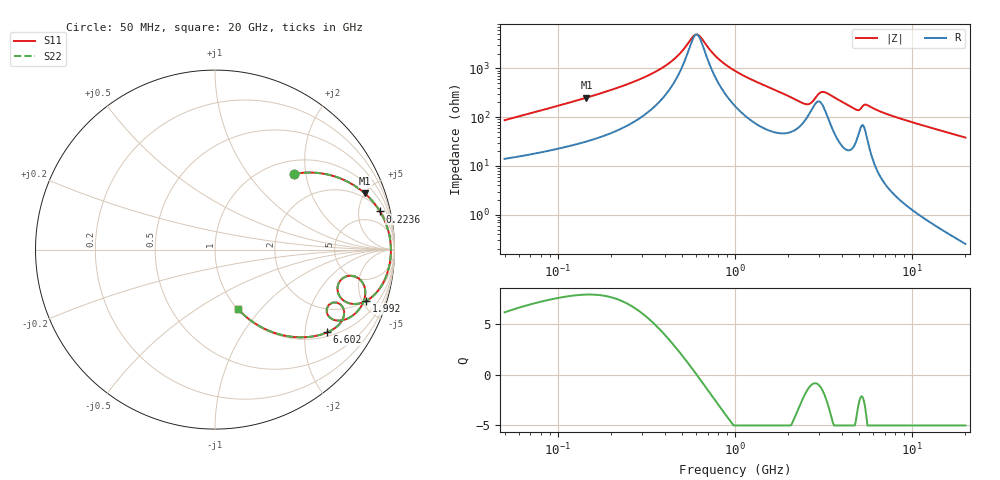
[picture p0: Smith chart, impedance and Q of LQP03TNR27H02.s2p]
!Murata Part Number: LQP03TNR27H02
!These Parameters are Measured in Series Mode Connection
!  o--[Z]--o
!Port1  Port2
!  o-------o
!Freq. Start=50[MHz] Stop=20[GHz], 401[Steps]
# Hz S RI R 50
!Freq.(Hz) S11(Real) S11(Imag) S21(Real) S21(Imag) S12(Real) S12(Imag) S22(Real) S22(Imag)
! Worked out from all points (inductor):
!   401 points, 50 MHz to 20 GHz, reference 50 ohm
!   read as one part in series: L = 268 nH near 51.52 MHz
!   highest Q = 7.85 at 144.8 MHz (marker M1), where L = 273 nH
!   self-resonance near 606.3 MHz
!   S11 on the Smith chart (normalised r, x): 50 MHz: 1.28, +1.71; 223.6 MHz: 2.13, +8.23; 1.992 GHz: 1.95, -5.37; 6.602 GHz: 1.12, -2.61; 20 GHz: 1.01, -0.76
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5e7  0.4391 0.4211  0.5609 -0.4211  0.5609 -0.4211  0.4391 0.4211
1.364002e8  0.8178 0.3274  0.1822 -0.3274  0.1822 -0.3274  0.8178 0.3274
1.448224e8  0.8337 0.3141  0.1663 -0.3141  0.1663 -0.3141  0.8337 0.3141
2.236068e8  0.9193 0.2124  0.0807 -0.2124  0.0807 -0.2124  0.9193 0.2124
3.721004e8  0.9672 0.0989  0.0328 -0.0989  0.0328 -0.0989  0.9672 0.0989
4.589149e8  0.9758 0.0558  0.0242 -0.0558  0.0242 -0.0558  0.9758 0.0558
6.100003e8  0.9802 -0.00121  0.0198 0.00121  0.0198 0.00121  0.9802 -0.00121
7.987718e8  0.9769 -0.0561  0.0231 0.0561  0.0231 0.0561  0.9769 -0.0561
1e9  0.9676 -0.1049  0.0324 0.1049  0.0324 0.1049  0.9676 -0.1049
1.99176e9  0.8429 -0.2858  0.1571 0.2858  0.1571 0.2858  0.8429 -0.2858
2.419936e9  0.7176 -0.2846  0.2824 0.2846  0.2824 0.2846  0.7176 -0.2846
2.728004e9  0.6972 -0.1736  0.3028 0.1736  0.3028 0.1736  0.6972 -0.1736
3.121702e9  0.8199 -0.1806  0.1801 0.1806  0.1801 0.1806  0.8199 -0.1806
3.680849e9  0.8206 -0.3052  0.1794 0.3052  0.1794 0.3052  0.8206 -0.3052
4.539627e9  0.6996 -0.3952  0.3004 0.3952  0.3004 0.3952  0.6996 -0.3952
4.966507e9  0.6226 -0.3493  0.3774 0.3493  0.3774 0.3493  0.6226 -0.3493
5.273168e9  0.6793 -0.295  0.3207 0.295  0.3207 0.295  0.6793 -0.295
5.683258e9  0.7154 -0.3782  0.2846 0.3782  0.2846 0.3782  0.7154 -0.3782
6.601595e9  0.6255 -0.4611  0.3745 0.4611  0.3745 0.4611  0.6255 -0.4611
7.442007e9  0.5512 -0.4827  0.4488 0.4827  0.4488 0.4827  0.5512 -0.4827
1.238412e10  0.2845 -0.4454  0.7155 0.4454  0.7155 0.4454  0.2845 -0.4454
2e10  0.1291 -0.3321  0.8709 0.3321  0.8709 0.3321  0.1291 -0.3321
